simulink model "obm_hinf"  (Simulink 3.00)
settings: Solver=ode5  StartTime=0.0  StopTime=20.0  FixedStep=Ts  RelTol=1e-3
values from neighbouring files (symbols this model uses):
  ac = 1-pc    [obm_sim_hinf.m]    (also in obm_sim_pid.m; obm_sim_smcrssi.m)
  coordinate_sw = 1    [obm_sim_hinf.m]    (also in obm_sim_pid.m; obm_sim_smcrssi.m)
  F = [66,24]    [obm_hinf_syn.m]    (also in obm_sim_hinf.m)
  lim1 = 262.5e-3    (= 0.2625)    [obm_sim_hinf.m]    (also in obm_sim_pid.m; obm_sim_smcrssi.m = 1.3125)
  lim2 = 26.9e-3    (= 0.0269)    [obm_sim_hinf.m]    (also in obm_sim_pid.m; obm_sim_smcrssi.m = 0.1345)
  oscillation_start = 10    [obm_sim_hinf.m]    (also in obm_sim_pid.m; obm_sim_smcrssi.m)
  p = zeros(1,12)    [obm_pset.m]
  pc = input('Choice of the problem: enter 0 for attitude or 1 for postion.')    [obm_sim_hinf.m]    (also in obm_sim_pid.m = input('Selection of the problem: enter 0 for attitude or 1 f; obm_sim_smcrssi.m)
  pn = zeros(1,12)    [obm_pnset.m]
  r0 = 5    [obm_sim_hinf.m]    (also in obm_sim_pid.m; obm_sim_smcrssi.m)
  step1 = 30    [obm_sim_hinf.m]    (also in obm_sim_pid.m; obm_sim_smcrssi.m)
  step2 = 90    [obm_sim_hinf.m]    (also in obm_sim_pid.m; obm_sim_smcrssi.m)
  sw = input('choice of the ocsillation type: enter 1 for single; 2 for double; 3 for Bretschneider.')    [obm_hinf_syn.m]    (also in obm_sim_hinf.m = input('Choice of the ocsillation type: enter 1 for single; 2; obm_sim_pid.m = input('Selection of the ocsillation type: enter 1 for single; obm_sim_smcrssi.m = input('Choice of the ocsillation type: enter 1 for single; 2)
  Ts = 0.01    [obm_sim_hinf.m]    (also in obm_sim_pid.m; obm_sim_smcrssi.m = 0.001)
  X = 0.06    [obm_sim_hinf.m]    (also in obm_sim_pid.m; obm_sim_smcrssi.m)
  xy0 = obm_kinematics([r0;r0]*pi/180,0)    [obm_sim_hinf.m]    (also in obm_sim_pid.m; obm_sim_smcrssi.m)
  Y = 0.13    [obm_sim_hinf.m]    (also in obm_sim_pid.m; obm_sim_smcrssi.m)
undefined symbols (not defined in the file or in its folder): A1d, akd, B1d, base_oscillation, bkd, C1d, ckd, D1d, dkd, obm_distH, obm_inv_kinematics, obm_kinematics, obm_M, obm_nlsfb1, obm_sys
libraries: simulink3 x2

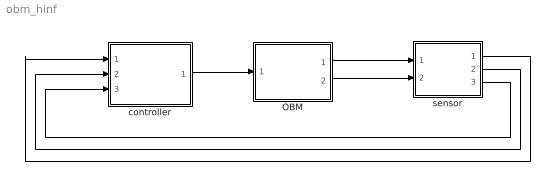
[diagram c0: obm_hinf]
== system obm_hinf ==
  OBM : Subsystem
  controller : Subsystem
  sensor : Subsystem
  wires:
  controller/1(control input) -> OBM/1(control input)
  OBM/1(q(t)) -> sensor/1(q(t))
  OBM/2(qb(t)) -> sensor/2(qb(t))
  sensor/1(qk) -> controller/1(qk)
  sensor/2(dqk) -> controller/2(dqk)
  sensor/3(qbk) -> controller/3(qbk)

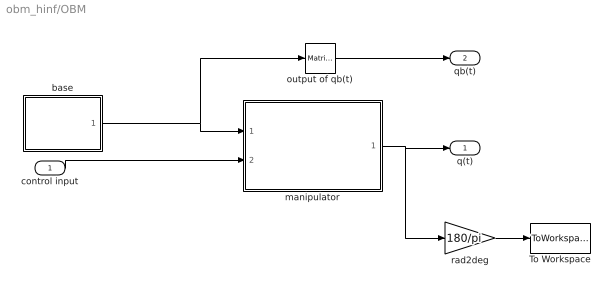
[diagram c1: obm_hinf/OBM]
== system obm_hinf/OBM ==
  control input : Inport  Port=1  PortWidth=-1  SampleTime=-1  DataType=auto
  To Workspace : ToWorkspace  VariableName=qout  SampleTime=-1  SaveFormat=Matrix
  base : Subsystem
  manipulator : Subsystem
  output of qb(t) : simulink3/Math/Matrix Gain  K=[1 0 0]
  rad2deg : Gain  Gain=180/pi  SaturateOnIntegerOverflow=on
  q(t) : Outport  Port=1
  qb(t) : Outport  Port=2
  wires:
  control input/1 -> manipulator/2(control input)
  base/1(oscillation) -> manipulator/1(base oscillation), output of qb(t)/1
  output of qb(t)/1 -> qb(t)/1
  rad2deg/1 -> To Workspace/1
  manipulator/1(q) -> q(t)/1, rad2deg/1

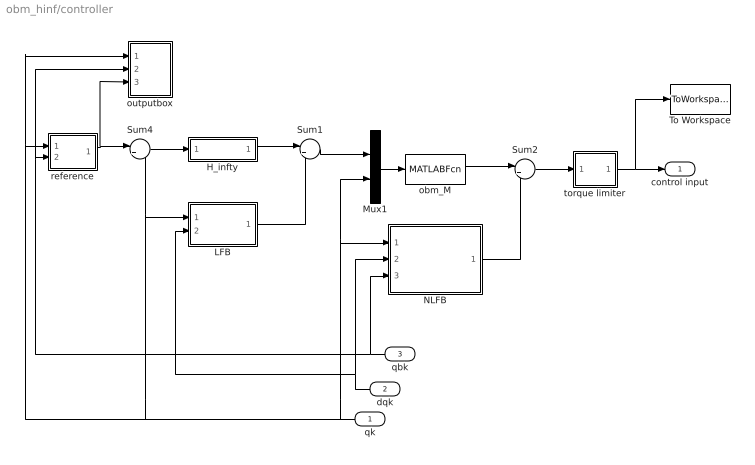
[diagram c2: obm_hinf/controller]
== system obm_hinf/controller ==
  qk : Inport  Orientation=left  Port=1  PortWidth=-1  SampleTime=-1  DataType=auto
  dqk : Inport  Orientation=left  Port=2  PortWidth=-1  SampleTime=-1  DataType=auto
  qbk : Inport  Orientation=left  Port=3  PortWidth=-1  SampleTime=-1  DataType=auto
  H_infty : Subsystem
  LFB : Subsystem
  Mux1 : Mux  Inputs=2
  NLFB : Subsystem
  Sum1 : Sum  Inputs=|++  SaturateOnIntegerOverflow=on
  Sum2 : Sum  Inputs=|++  SaturateOnIntegerOverflow=on
  Sum4 : Sum  Inputs=|+-  SaturateOnIntegerOverflow=on
  To Workspace : ToWorkspace  VariableName=torque  SampleTime=-1  SaveFormat=Matrix
  obm_M : MATLABFcn  MATLABFcn=obm_M([u(3);u(4)],pn,[u(1);u(2)])  OutputWidth=2  OutputSignalType=auto
  outputbox : Subsystem
  reference : Subsystem
  torque limiter : Subsystem
  control input : Outport  Port=1
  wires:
  Sum2/1 -> torque limiter/1(In)
  Mux1/1 -> obm_M/1
  obm_M/1 -> Sum2/1
  NLFB/1(nlfb) -> Sum2/2
  qk/1 -> Sum4/2, LFB/1(qk), outputbox/1(qk), reference/1(qk), Mux1/2, NLFB/1(qk)
  dqk/1 -> LFB/2(dqk), NLFB/2(dqk)
  qbk/1 -> NLFB/3(qbk), outputbox/2(qbk), reference/2(qbk)
  torque limiter/1(Out) -> control input/1, To Workspace/1
  H_infty/1(u) -> Sum1/1
  LFB/1(lfb) -> Sum1/2
  Sum1/1 -> Mux1/1
  Sum4/1 -> H_infty/1(e)
  reference/1(r) -> Sum4/1, outputbox/3(r)

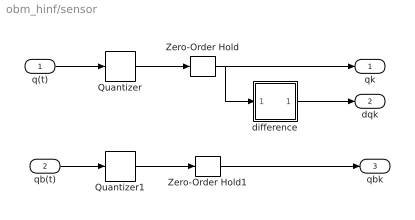
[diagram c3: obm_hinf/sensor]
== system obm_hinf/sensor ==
  q(t) : Inport  Port=1  PortWidth=-1  SampleTime=-1  DataType=auto
  qb(t) : Inport  Port=2  PortWidth=-1  SampleTime=-1  DataType=auto
  Quantizer : Quantizer  QuantizationInterval=rslv
  Quantizer1 : Quantizer  QuantizationInterval=rslv
  Zero-Order Hold : ZeroOrderHold  SampleTime=Ts
  Zero-Order Hold1 : ZeroOrderHold  SampleTime=Ts
  difference : Subsystem
  qk : Outport  Port=1
  dqk : Outport  Port=2
  qbk : Outport  Port=3
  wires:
  difference/1(Out1) -> dqk/1
  q(t)/1 -> Quantizer/1
  Quantizer/1 -> Zero-Order Hold/1
  Zero-Order Hold/1 -> qk/1, difference/1(In1)
  qb(t)/1 -> Quantizer1/1
  Quantizer1/1 -> Zero-Order Hold1/1
  Zero-Order Hold1/1 -> qbk/1

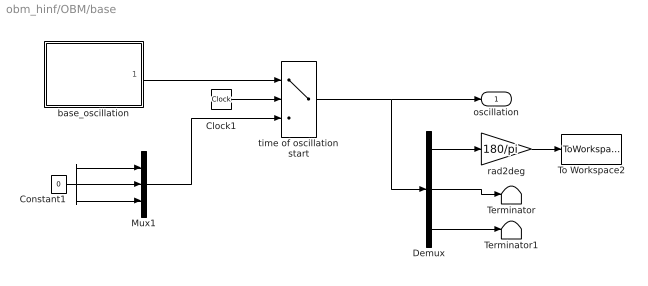
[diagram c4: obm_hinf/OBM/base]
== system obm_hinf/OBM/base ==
  Clock1 : Clock
  Constant1 : Constant  Value=0
  Demux : Demux  Outputs=3
  Mux1 : Mux  Inputs=3
  Terminator : Terminator
  Terminator1 : Terminator
  To Workspace2 : ToWorkspace  VariableName=qbout  SampleTime=-1  SaveFormat=Matrix
  base_oscillation : Subsystem
  rad2deg : Gain  Gain=180/pi  SaturateOnIntegerOverflow=on
  time of oscillation start : Switch  Threshold=oscillation_start
  oscillation : Outport  Port=1
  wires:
  Mux1/1 -> time of oscillation start/3
  Constant1/1 -> Mux1/2, Mux1/1, Mux1/3
  time of oscillation start/1 -> Demux/1, oscillation/1
  Demux/2 -> Terminator/1
  Demux/3 -> Terminator1/1
  Demux/1 -> rad2deg/1
  rad2deg/1 -> To Workspace2/1
  Clock1/1 -> time of oscillation start/2
  base_oscillation/1(base_oscilation) -> time of oscillation start/1

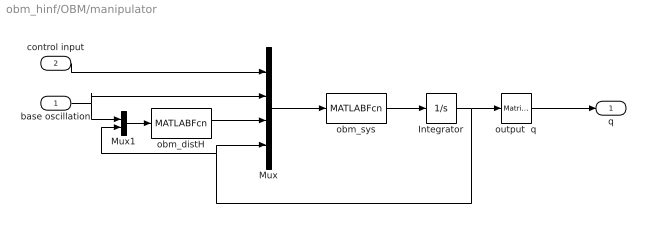
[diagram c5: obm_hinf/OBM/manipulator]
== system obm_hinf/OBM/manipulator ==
  base oscillation : Inport  Port=1  PortWidth=-1  SampleTime=-1  DataType=auto
  control input : Inport  Port=2  PortWidth=-1  SampleTime=-1  DataType=auto
  Integrator : Integrator  ExternalReset=none  InitialConditionSource=internal  InitialCondition=0  LimitOutput=off  UpperSaturationLimit=inf  LowerSaturationLimit=-inf  ShowSaturationPort=off  ShowStatePort=off  AbsoluteTolerance=auto
  Mux : Mux  Inputs=4
  Mux1 : Mux  Inputs=2
  obm_distH : MATLABFcn  MATLABFcn=obm_distH([u(4);u(5);u(6);u(7)],[u(1);u(2);u(3)],p)  OutputWidth=2  OutputSignalType=auto
  obm_sys : MATLABFcn  MATLABFcn=obm_sys([u(8);u(9);u(10);u(11)],[u(1);u(2)],u(3),[u(6);u(7)],p)  OutputWidth=4  OutputSignalType=auto
  output  q : simulink3/Math/Matrix Gain  K=[1 0 0 0; 0 1 0 0]
  q : Outport  Port=1
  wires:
  Mux1/1 -> obm_distH/1
  Mux/1 -> obm_sys/1
  obm_distH/1 -> Mux/3
  control input/1 -> Mux/1
  obm_sys/1 -> Integrator/1
  Integrator/1 -> output  q/1, Mux/4, Mux1/2
  base oscillation/1 -> Mux/2, Mux1/1
  output  q/1 -> q/1

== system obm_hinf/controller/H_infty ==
  e : Inport  Port=1  PortWidth=-1  SampleTime=-1  DataType=auto
  Discrete State-Space : DiscreteStateSpace  A=akd  B=bkd  C=ckd  D=dkd  X0=0  SampleTime=Ts
  Gain1 : Gain  Gain=-1  SaturateOnIntegerOverflow=on
  To Workspace6 : ToWorkspace  VariableName=eout  SampleTime=-1  SaveFormat=Matrix
  To Workspace7 : ToWorkspace  VariableName=hout  SampleTime=-1  SaveFormat=Matrix
  u : Outport  Port=1
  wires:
  e/1 -> Gain1/1
  Gain1/1 -> Discrete State-Space/1, To Workspace6/1
  Discrete State-Space/1 -> u/1, To Workspace7/1

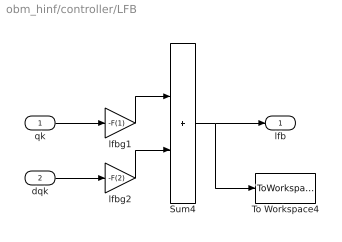
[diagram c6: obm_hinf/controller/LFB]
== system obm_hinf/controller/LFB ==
  qk : Inport  Port=1  PortWidth=-1  SampleTime=-1  DataType=auto
  dqk : Inport  Port=2  PortWidth=-1  SampleTime=-1  DataType=auto
  Sum4 : Sum  Inputs=|++  SaturateOnIntegerOverflow=on
  To Workspace4 : ToWorkspace  VariableName=pdout  SampleTime=-1  SaveFormat=Matrix
  lfbg1 : Gain  Gain=-F(1)  SaturateOnIntegerOverflow=on
  lfbg2 : Gain  Gain=-F(2)  SaturateOnIntegerOverflow=on
  lfb : Outport  Port=1
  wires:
  lfbg1/1 -> Sum4/1
  qk/1 -> lfbg1/1
  dqk/1 -> lfbg2/1
  lfbg2/1 -> Sum4/2
  Sum4/1 -> lfb/1, To Workspace4/1

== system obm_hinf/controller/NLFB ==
  qk : Inport  Port=1  PortWidth=-1  SampleTime=-1  DataType=auto
  dqk : Inport  Port=2  PortWidth=-1  SampleTime=-1  DataType=auto
  qbk : Inport  Port=3  PortWidth=-1  SampleTime=-1  DataType=auto
  Mux1 : Mux  Inputs=3
  obm_nlsfb1 : MATLABFcn  MATLABFcn=obm_nlsfb1([u(1);u(2);u(3);u(4)],u(5),pn)  OutputWidth=2  OutputSignalType=auto
  nlfb : Outport  Port=1
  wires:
  Mux1/1 -> obm_nlsfb1/1
  qk/1 -> Mux1/1
  qbk/1 -> Mux1/3
  dqk/1 -> Mux1/2
  obm_nlsfb1/1 -> nlfb/1

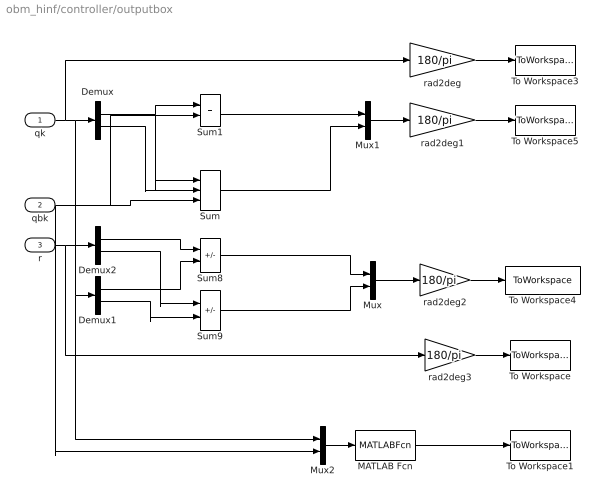
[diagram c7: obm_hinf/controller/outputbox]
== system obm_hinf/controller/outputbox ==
  qk : Inport  Port=1  PortWidth=-1  SampleTime=-1  DataType=auto
  qbk : Inport  Port=2  PortWidth=-1  SampleTime=-1  DataType=auto
  r : Inport  Port=3  PortWidth=-1  SampleTime=-1  DataType=auto
  Demux : Demux  Outputs=2
  Demux1 : Demux  Outputs=2
  Demux2 : Demux  Outputs=2
  MATLAB Fcn : MATLABFcn  MATLABFcn=norm(obm_kinematics([u(1);u(2)],u(3))-[X;Y])  OutputWidth=1  OutputSignalType=auto
  Mux : Mux  Inputs=2
  Mux1 : Mux  Inputs=2
  Mux2 : Mux  Inputs=2
  Sum : Sum  Inputs=|+++  SaturateOnIntegerOverflow=on
  Sum1 : Sum  Inputs=|++  SaturateOnIntegerOverflow=on
  Sum8 : Sum  Inputs=|+-  SaturateOnIntegerOverflow=on
  Sum9 : Sum  Inputs=|+-  SaturateOnIntegerOverflow=on
  To Workspace : ToWorkspace  VariableName=rqout  SampleTime=-1  SaveFormat=Matrix
  To Workspace1 : ToWorkspace  VariableName=xyout  SampleTime=-1  SaveFormat=Matrix
  To Workspace3 : ToWorkspace  VariableName=qkout  SampleTime=-1  SaveFormat=Matrix
  To Workspace4 : ToWorkspace  VariableName=qkerror_out  SampleTime=Ts  SaveFormat=Matrix
  To Workspace5 : ToWorkspace  VariableName=gqkout  SampleTime=-1  SaveFormat=Matrix
  rad2deg{,1..3} (4 alike) : Gain  Gain=180/pi  SaturateOnIntegerOverflow=on
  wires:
  qk/1 -> rad2deg/1, Demux/1, Demux1/1, Mux2/1
  Mux1/1 -> rad2deg1/1
  Demux/2 -> Sum/2
  Sum1/1 -> Mux1/1
  rad2deg1/1 -> To Workspace5/1
  rad2deg/1 -> To Workspace3/1
  Sum/1 -> Mux1/2
  Demux2/1 -> Sum8/1
  Demux2/2 -> Sum9/1
  Demux1/2 -> Sum9/2
  Sum8/1 -> Mux/1
  Sum9/1 -> Mux/2
  Mux/1 -> rad2deg2/1
  Demux1/1 -> Sum8/2
  rad2deg2/1 -> To Workspace4/1
  Demux/1 -> Sum1/1, Sum/1
  rad2deg3/1 -> To Workspace/1
  r/1 -> Demux2/1, rad2deg3/1
  Mux2/1 -> MATLAB Fcn/1
  qbk/1 -> Sum/3, Sum1/2, Mux2/2
  MATLAB Fcn/1 -> To Workspace1/1

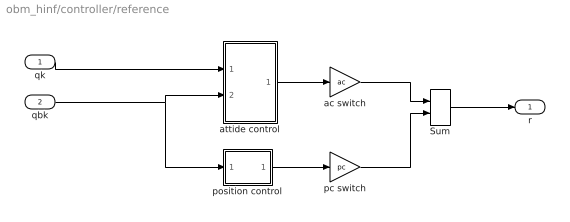
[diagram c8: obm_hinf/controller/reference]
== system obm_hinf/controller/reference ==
  qk : Inport  Port=1  PortWidth=-1  SampleTime=-1  DataType=auto
  qbk : Inport  Port=2  PortWidth=-1  SampleTime=-1  DataType=auto
  Sum : Sum  Inputs=|++  SaturateOnIntegerOverflow=on
  ac switch : Gain  Gain=ac  SaturateOnIntegerOverflow=on
  attide control : Subsystem
  pc switch : Gain  Gain=pc  SaturateOnIntegerOverflow=on
  position control : Subsystem
  r : Outport  Port=1
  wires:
  qk/1 -> attide control/1(In1)
  qbk/1 -> attide control/2(In2), position control/1(qbk)
  attide control/1(Out1) -> ac switch/1
  position control/1(r2) -> pc switch/1
  ac switch/1 -> Sum/1
  pc switch/1 -> Sum/2
  Sum/1 -> r/1

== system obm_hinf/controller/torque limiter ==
  In : Inport  Port=1  PortWidth=-1  SampleTime=-1  DataType=auto
  Demux1 : Demux  Outputs=2
  Mux1 : Mux  Inputs=2
  Saturation : Saturate  UpperLimit=lim1  LowerLimit=-lim1
  Saturation1 : Saturate  UpperLimit=lim2  LowerLimit=-lim2
  To Workspace1 : ToWorkspace  VariableName=torout2  SampleTime=-1  SaveFormat=Matrix
  Out : Outport  Port=1
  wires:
  Saturation/1 -> Mux1/1
  Demux1/1 -> Saturation/1
  Demux1/2 -> Saturation1/1
  Saturation1/1 -> Mux1/2
  In/1 -> Demux1/1
  Mux1/1 -> Out/1, To Workspace1/1

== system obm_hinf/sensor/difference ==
  In1 : Inport  Port=1  PortWidth=-1  SampleTime=-1  DataType=auto
  Gain12 : Gain  Gain=1/Ts  SaturateOnIntegerOverflow=on
  Sum23 : Sum  Inputs=|-+  SaturateOnIntegerOverflow=on
  Unit Delay5 : UnitDelay  X0=0  SampleTime=Ts
  Out1 : Outport  Port=1
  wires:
  Gain12/1 -> Out1/1
  Unit Delay5/1 -> Sum23/1
  Sum23/1 -> Gain12/1
  In1/1 -> Unit Delay5/1, Sum23/2

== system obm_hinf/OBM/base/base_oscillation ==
  Clock3 : Clock
  Derivative6 : Derivative
  Derivative7 : Derivative
  Mux4 : Mux  Inputs=3
  base_oscillation : MATLABFcn  MATLABFcn=base_oscillation(u,sw)  OutputWidth=-1  OutputSignalType=auto
  base_oscilation : Outport  Port=1
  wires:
  Clock3/1 -> base_oscillation/1
  Derivative6/1 -> Mux4/3
  Derivative7/1 -> Mux4/2, Derivative6/1
  base_oscillation/1 -> Mux4/1, Derivative7/1
  Mux4/1 -> base_oscilation/1

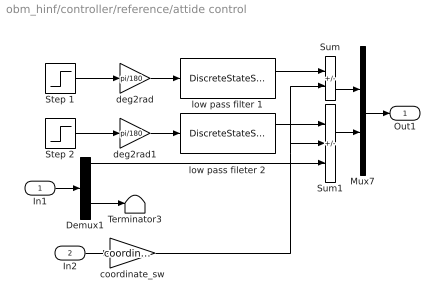
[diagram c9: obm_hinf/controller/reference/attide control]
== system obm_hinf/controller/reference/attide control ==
  In1 : Inport  Port=1  PortWidth=-1  SampleTime=-1  DataType=auto
  In2 : Inport  Port=2  PortWidth=-1  SampleTime=-1  DataType=auto
  Demux1 : Demux  Outputs=2
  Mux7 : Mux  Inputs=2
  Step 1 : Step  Time=10  Before=0  After=step1  SampleTime=Ts
  Step 2 : Step  Time=10  Before=0  After=step2  SampleTime=Ts
  Sum : Sum  Inputs=|+-  SaturateOnIntegerOverflow=on
  Sum1 : Sum  Inputs=|+--  SaturateOnIntegerOverflow=on
  Terminator3 : Terminator
  coordinate_sw : Gain  Gain=coordinate_sw  SaturateOnIntegerOverflow=on
  deg2rad : Gain  Gain=pi/180  SaturateOnIntegerOverflow=on
  deg2rad1 : Gain  Gain=pi/180  SaturateOnIntegerOverflow=on
  low pass fileter 2 : DiscreteStateSpace  A=A1d  B=B1d  C=C1d  D=D1d  X0=0  SampleTime=Ts
  low pass filter 1 : DiscreteStateSpace  A=A1d  B=B1d  C=C1d  D=D1d  X0=0  SampleTime=Ts
  Out1 : Outport  Port=1
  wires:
  Sum/1 -> Mux7/1
  Sum1/1 -> Mux7/2
  low pass filter 1/1 -> Sum/1
  low pass fileter 2/1 -> Sum1/1
  Demux1/2 -> Terminator3/1
  Demux1/1 -> Sum1/3
  coordinate_sw/1 -> Sum/2, Sum1/2
  deg2rad/1 -> low pass filter 1/1
  Step 1/1 -> deg2rad/1
  deg2rad1/1 -> low pass fileter 2/1
  Step 2/1 -> deg2rad1/1
  Mux7/1 -> Out1/1
  In1/1 -> Demux1/1
  In2/1 -> coordinate_sw/1

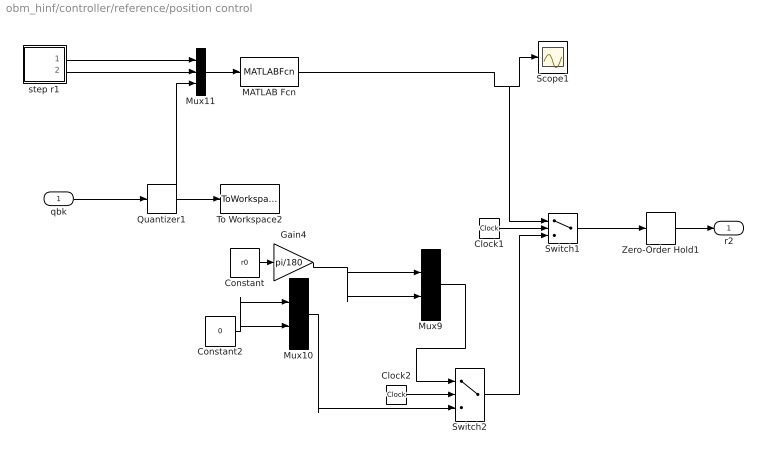
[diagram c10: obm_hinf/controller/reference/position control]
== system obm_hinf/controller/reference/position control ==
  qbk : Inport  Port=1  PortWidth=-1  SampleTime=-1  DataType=auto
  Clock1 : Clock
  Clock2 : Clock
  Constant : Constant  Value=r0
  Constant2 : Constant  Value=0
  Gain4 : Gain  Gain=pi/180  SaturateOnIntegerOverflow=on
  MATLAB Fcn : MATLABFcn  MATLABFcn=obm_inv_kinematics([u(1);u(2)],u(3))  OutputWidth=2  OutputSignalType=auto
  Mux10 : Mux  Inputs=2
  Mux11 : Mux  Inputs=3
  Mux9 : Mux  Inputs=2
  Quantizer1 : Quantizer  QuantizationInterval=rslv
  Scope1 : Scope
  Switch1 : Switch  Threshold=6
  Switch2 : Switch  Threshold=4
  To Workspace2 : ToWorkspace  VariableName=baseout2  SampleTime=-1  SaveFormat=Matrix
  Zero-Order Hold1 : ZeroOrderHold  SampleTime=Ts
  step r1 : Subsystem
  r2 : Outport  Port=1
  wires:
  Clock1/1 -> Switch1/2
  Clock2/1 -> Switch2/2
  Constant2/1 -> Mux10/2, Mux10/1
  Constant/1 -> Gain4/1
  Switch2/1 -> Switch1/3
  Mux9/1 -> Switch2/1
  Mux10/1 -> Switch2/3
  Gain4/1 -> Mux9/2, Mux9/1
  Zero-Order Hold1/1 -> r2/1
  Switch1/1 -> Zero-Order Hold1/1
  Quantizer1/1 -> To Workspace2/1, Mux11/3
  Mux11/1 -> MATLAB Fcn/1
  MATLAB Fcn/1 -> Scope1/1, Switch1/1
  step r1/1(x) -> Mux11/1
  step r1/2(y) -> Mux11/2
  qbk/1 -> Quantizer1/1

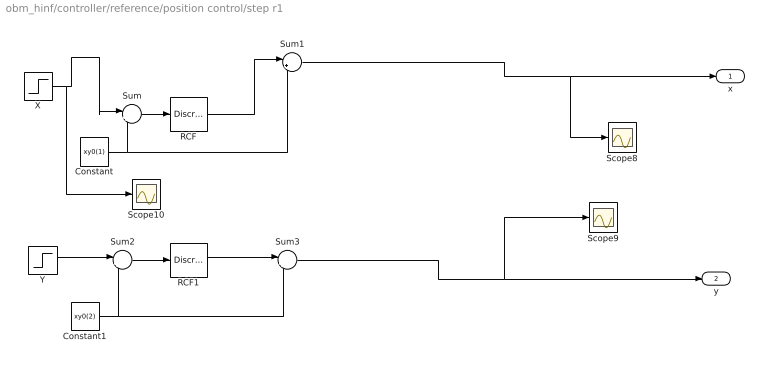
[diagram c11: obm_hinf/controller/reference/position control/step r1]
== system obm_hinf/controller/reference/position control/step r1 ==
  Constant : Constant  Value=xy0(1)
  Constant1 : Constant  Value=xy0(2)
  RCF : DiscreteStateSpace  A=A1d  B=B1d  C=C1d  D=D1d  X0=0  SampleTime=Ts
  RCF1 : DiscreteStateSpace  A=A1d  B=B1d  C=C1d  D=D1d  X0=0  SampleTime=Ts
  Scope10 : Scope
  Scope8 : Scope
  Scope9 : Scope
  Sum : Sum  Inputs=|+-  SaturateOnIntegerOverflow=on
  Sum1 : Sum  Inputs=|++  SaturateOnIntegerOverflow=on
  Sum2 : Sum  Inputs=|+-  SaturateOnIntegerOverflow=on
  Sum3 : Sum  Inputs=|++  SaturateOnIntegerOverflow=on
  X : Step  Time=6  Before=xy0(1)  After=X  SampleTime=0
  Y : Step  Time=6  Before=xy0(2)  After=Y  SampleTime=0
  x : Outport  Port=1
  y : Outport  Port=2
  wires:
  X/1 -> Scope10/1, Sum/1
  Sum1/1 -> x/1, Scope8/1
  Sum/1 -> RCF/1
  RCF/1 -> Sum1/1
  Constant/1 -> Sum/2, Sum1/2
  Y/1 -> Sum2/1
  Sum2/1 -> RCF1/1
  Constant1/1 -> Sum2/2, Sum3/2
  RCF1/1 -> Sum3/1
  Sum3/1 -> y/1, Scope9/1
